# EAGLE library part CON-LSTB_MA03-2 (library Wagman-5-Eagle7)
PIN HEADER
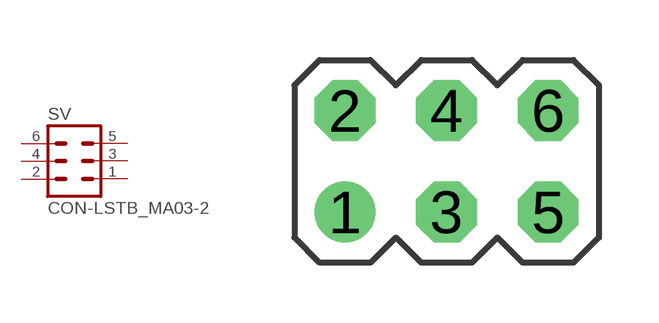
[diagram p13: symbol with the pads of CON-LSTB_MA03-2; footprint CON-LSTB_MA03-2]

Designator prefix SV

## CON-LSTB_MA03-2 (OC_FARNELL: unknown; OC_NEWARK: unknown)  [CON-LSTB_MA03-2]
1  1  pas
2  2  pas
3  3  pas
4  4  pas
5  5  pas
6  6  pas

## Footprint CON-LSTB_MA03-2 (pad centres in mm)
PIN HEADER
drill 1.016: 1 -2.54,-1.27
drill 1.016 octagon: 2 -2.54,1.27; 3 0,-1.27; 4 0,1.27; 5 2.54,-1.27; 6 2.54,1.27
